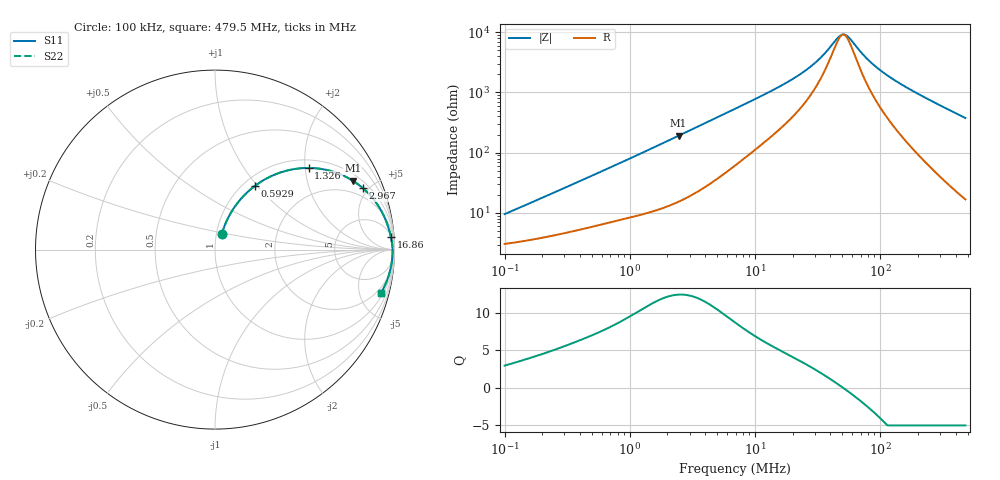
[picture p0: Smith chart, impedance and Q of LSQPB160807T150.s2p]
! LSQPB160807T150  S-PARAMETER MODEL  ( General Type )
! Model Generated by TAIYO YUDEN Corporation (http://www.ty-top.com)
! Version 1.0
! TAIYO YUDEN Control No. 110308NG25SB-FKC
! Copyright(c) 2011 TAIYO YUDEN CO.,LTD. All Rights Reserved.
! Product Description (link to TY-COMPAS)
! https://ds.yuden.co.jp/TYCOMPAS/or/detail?pn=LSQPB160807T150M&u=M
! Products Name : Inductors
! Characteristics :
!  Inductance : 15 uH , SRF(min) : 32 MHz , DC Resistance(max) : 3.328 Ohm
!  Rated Current : Saturation :150 mA , Temp Rise : 200 mA (40 degC)
!  Case Size : 1.6 x 0.8 / 0.063 x 0.031 [mm/inch] , Thickness : 0.7 / 0.028 [mm/inch]
!  (Conditions: Temperature = 25 degC , DC Bias Current/Voltage = 0A / 0V)
! External Node Assignments :
!  1  o---GGG---o  2
! GND o---------o GND
! Frequency Range : 0.1MHz  -  479.524407MHz  [ 402 STEP ]
# MHz S RI R 50
! Freq[MHz].  S11 Real  S11 Imag  S21 Real  S21 Imag  S12 Real  S12 Imag  S22 Real  S22 Imag
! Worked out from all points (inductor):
!   401 points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, 100 kHz to 479.5 MHz, reference 50 ohm
!   read as one part in series: L = 14.3 uH near 104.3 kHz
!   highest Q = 12.4 at 2.452 MHz (marker M1), where L = 12.4 uH
!   self-resonance near 50.65 MHz
!   S11 on the Smith chart (normalised r, x): 100 kHz: 1.06, +0.18; 592.9 kHz: 1.13, +0.97; 1.326 MHz: 1.20, +2.09; 2.967 MHz: 1.37, +4.60; 16.86 MHz: 7, +27; 479.5 MHz: 1.34, -7.53
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0.1  0.0372 0.0848  0.9628 -0.0848  0.9628 -0.0848  0.0372 0.0848
0.228496  0.073 0.1764  0.927 -0.1764  0.927 -0.1764  0.073 0.1764
0.413557  0.143 0.2809  0.857 -0.2809  0.857 -0.2809  0.143 0.2809
0.592885  0.2218 0.3544  0.7782 -0.3544  0.7782 -0.3544  0.2218 0.3544
0.925151  0.3694 0.4312  0.6306 -0.4312  0.6306 -0.4312  0.3694 0.4312
1.326317  0.5219 0.455  0.4781 -0.455  0.4781 -0.455  0.5219 0.455
1.710297  0.6324 0.4413  0.3676 -0.4413  0.3676 -0.4413  0.6324 0.4413
2.451919  0.7674 0.3841  0.2326 -0.3841  0.2326 -0.3841  0.7674 0.3841
2.967046  0.8227 0.3434  0.1773 -0.3434  0.1773 -0.3434  0.8227 0.3434
4.43775  0.9024 0.2548  0.0976 -0.2548  0.0976 -0.2548  0.9024 0.2548
7.073061  0.9492 0.169  0.0508 -0.169  0.0508 -0.169  0.9492 0.169
16.86128  0.9801 0.0696  0.0199 -0.0696  0.0199 -0.0696  0.9801 0.0696
22.68396  0.9844 0.0475  0.0156 -0.0475  0.0156 -0.0475  0.9844 0.0475
28.6379  0.9866 0.0324  0.0134 -0.0324  0.0134 -0.0324  0.9866 0.0324
35.39659  0.988 0.0199  0.012 -0.0199  0.012 -0.0199  0.988 0.0199
46.62166  0.989 0.00455  0.011 -0.00455  0.011 -0.00455  0.989 0.00455
51.83199  0.9892 -0.00127  0.0108 0.00127  0.0108 0.00127  0.9892 -0.00127
56.41648  0.9893 -0.00595  0.0107 0.00595  0.0107 0.00595  0.9893 -0.00595
82.61188  0.9889 -0.0281  0.0111 0.0281  0.0111 0.0281  0.9889 -0.0281
118.4342  0.987 -0.0528  0.013 0.0528  0.013 0.0528  0.987 -0.0528
218.9453  0.9769 -0.1119  0.0231 0.1119  0.0231 0.1119  0.9769 -0.1119
479.5244  0.9249 -0.2422  0.0751 0.2422  0.0751 0.2422  0.9249 -0.2422
